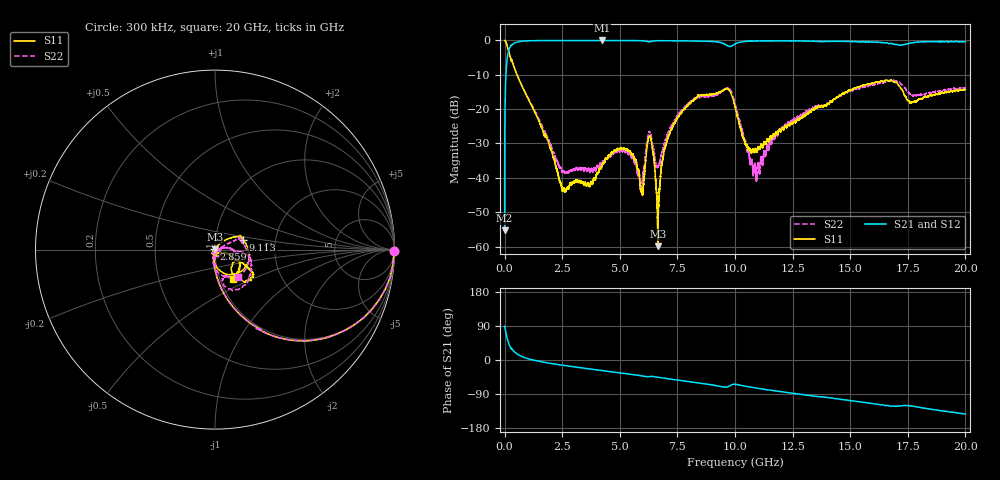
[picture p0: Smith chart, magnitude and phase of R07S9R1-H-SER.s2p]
!{R07S9R1}
!Johanson Technology Inc.
!www.johansontechnology.com
!Test Board Conditions:
!Substrate Type  RO4350B
!Substrate Thickness  10 mil
!Substrate Dk  3.66
!TL Type: GCPW
!TL Trace Width  21 mil
!TL Gap  20 mil
!Electrode orientation  Horizontal
!DUT TOPOLOGY	SERIES
!Mounting Pad LxW  16x21 mil
! Created Sat Feb  6 11:41:31 2021
# hz S ma R 50
! 2 Port Network Data from SP1.SP block
! freq  magS11  angS11  magS21  angS21  magS12  angS12  magS22  angS22
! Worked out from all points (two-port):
!   20001 points, 300 kHz to 20 GHz, reference 50 ohm
!   highest |S21| = -0.01 dB at 4.231 GHz (marker M1); lowest = -55.3 dB at 300 kHz (marker M2)
!   |S21| within 3 dB of the highest: 174.3 MHz to end of sweep
!   lowest |S11| = -59.9 dB at 6.653 GHz (marker M3), VSWR 1.00, Z = 49.9 + j0.0602 ohm
!   |S11| at or under -10 dB: 539.5 MHz to end of sweep
!   |S22| runs from -44.2 to 0.0 dB; largest |S21 - S12| = 0.014
!   S11 on the Smith chart (normalised r, x): 300 kHz: open; 2.859 GHz: 0.99, +0.01; 9.113 GHz: 1.36, +0.14; 20 GHz: 1.15, -0.40
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300000  0.9968 -0.4  0.001727 89.2  0.001787 90.7  0.9976 -0.4
1.073e8  0.8478 -32.3  0.5244 58.0  0.5251 58.0  0.8494 -32.2
2.563e8  0.5538 -57.9  0.8269 32.6  0.8257 32.7  0.5557 -57.9
7.773e8  0.2087 -81.7  0.9766 8.4  0.9768 8.4  0.2103 -81.1
2.4643e9  0.00785 -153.9  0.9975 -13.4  0.9971 -13.4  0.01313 -50.9
2.8593e9  0.008323 141.1  0.9968 -16.8  0.9973 -16.8  0.01287 -14.9
3.3343e9  0.008511 140.2  0.9972 -20.7  0.9975 -20.7  0.01299 -15.7
4.2313e9  0.01544 -137.4  0.9986 -27.9  0.997 -27.9  0.01603 -84.6
5.3623e9  0.02445 -124.6  0.9954 -36.8  0.9953 -36.9  0.02219 -121.3
5.9623e9  0.006506 -84.2  0.9905 -42.0  0.9902 -42.0  0.008439 -57.4
6.3033e9  0.04029 -59.3  0.9527 -43.3  0.9531 -43.3  0.04598 -54.3
6.6533e9  0.001012 143.4  0.9901 -45.6  0.9902 -45.7  0.01436 -32.0
6.6673e9  0.002861 88.4  0.99 -45.7  0.9898 -45.8  0.01482 -24.0
6.8963e9  0.02148 59.2  0.9922 -47.8  0.993 -47.8  0.02812 12.4
7.2993e9  0.05564 47.7  0.9911 -51.2  0.9904 -51.3  0.06126 23.4
9.1133e9  0.1653 18.1  0.9603 -67.0  0.9608 -67.0  0.1574 12.8
1.00003e10  0.1092 -80.9  0.8863 -63.9  0.8875 -63.9  0.121 -84.8
1.08643e10  0.02547 -54.5  0.9814 -73.6  0.9803 -73.5  0.01535 -49.6
1.33343e10  0.09481 -20.6  0.9761 -94.6  0.9769 -94.6  0.1016 -2.6
1.66673e10  0.2561 -37.0  0.902 -120.5  0.9065 -121.0  0.256 -45.2
1.76603e10  0.1264 -36.1  0.9208 -121.4  0.9234 -121.5  0.1671 -72.3
2e10  0.194 -58.6  0.9617 -142.6  0.9544 -142.6  0.2031 -50.0
